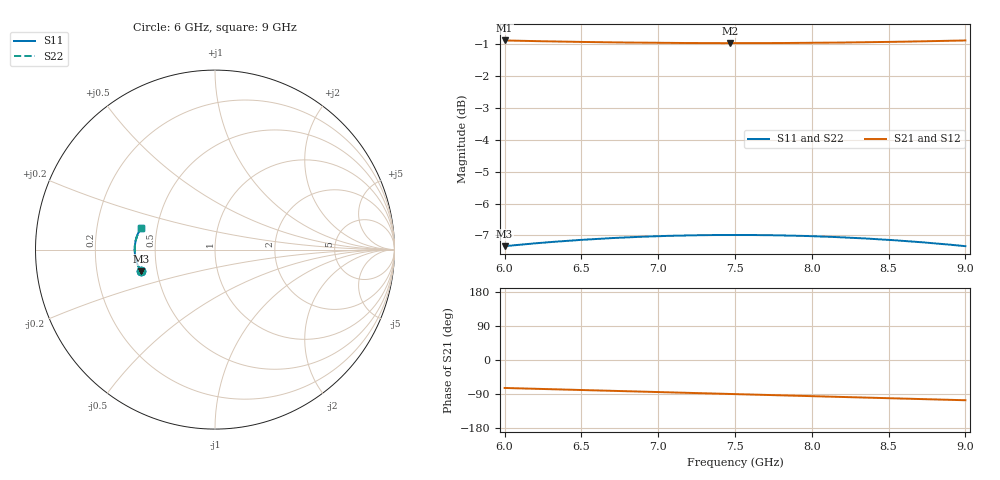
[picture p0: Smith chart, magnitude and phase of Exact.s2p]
!AWR Design Environment (2469) Mon Oct 04 18:05:22 2004
!freq-unit  param-type  data-format  keyword  impedance-ohms
# GHz  S  MA  R  50
!Freq  MagS11  AngS11  MagS21  AngS21  MagS12  AngS12  MagS22  AngS22
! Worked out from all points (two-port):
!   301 points, 6 GHz to 9 GHz, reference 50 ohm
!   highest |S21| = -0.89 dB at 6 GHz (marker M1); lowest = -1.0 dB at 7.47 GHz (marker M2)
!   |S21| within 3 dB of the highest: start of sweep to end of sweep
!   lowest |S11| = -7.3 dB at 6 GHz (marker M3), VSWR 2.51, Z = 20.3 - j5.96 ohm
!   |S11| at or under -10 dB: nowhere
!   |S22| runs from -7.3 to -7.0 dB; largest |S21 - S12| = 0
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6  0.4298 -163.8  0.9029 -73.8  0.9029 -73.8  0.4298 -163.8
6.25  0.4352 -166.5  0.9003 -76.5  0.9003 -76.5  0.4352 -166.5
6.38  0.4377 -167.9  0.8991 -77.9  0.8991 -77.9  0.4377 -167.9
6.5  0.4397 -169.2  0.8982 -79.2  0.8982 -79.2  0.4397 -169.2
6.62  0.4415 -170.5  0.8973 -80.5  0.8973 -80.5  0.4415 -170.5
6.75  0.4431 -171.9  0.8965 -81.9  0.8965 -81.9  0.4431 -171.9
6.89  0.4446 -173.4  0.8957 -83.4  0.8957 -83.4  0.4446 -173.4
7  0.4456 -174.6  0.8952 -84.6  0.8952 -84.6  0.4456 -174.6
7.23  0.447 -177.1  0.8945 -87.1  0.8945 -87.1  0.447 -177.1
7.47  0.4475 -179.7  0.8943 -89.7  0.8943 -89.7  0.4475 -179.7
7.5  0.4476 -180.0  0.8943 -90.0  0.8943 -90.0  0.4476 -180.0
7.62  0.4474 178.7  0.8943 -91.3  0.8943 -91.3  0.4474 178.7
7.75  0.4471 177.3  0.8945 -92.7  0.8945 -92.7  0.4471 177.3
7.87  0.4465 176.0  0.8948 -94.0  0.8948 -94.0  0.4465 176.0
8  0.4456 174.6  0.8952 -95.4  0.8952 -95.4  0.4456 174.6
8.11  0.4446 173.4  0.8957 -96.6  0.8957 -96.6  0.4446 173.4
8.25  0.4431 171.9  0.8965 -98.1  0.8965 -98.1  0.4431 171.9
8.38  0.4415 170.5  0.8973 -99.5  0.8973 -99.5  0.4415 170.5
8.5  0.4397 169.2  0.8982 -100.8  0.8982 -100.8  0.4397 169.2
8.62  0.4377 167.9  0.8991 -102.1  0.8991 -102.1  0.4377 167.9
8.75  0.4352 166.5  0.9003 -103.5  0.9003 -103.5  0.4352 166.5
9  0.4298 163.8  0.9029 -106.2  0.9029 -106.2  0.4298 163.8
